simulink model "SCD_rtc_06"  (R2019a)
settings: configuration reference "configurationSettings" (kept in a data dictionary, not in this file)
undefined symbols (not defined in the file or in its folder): algo_demo1_fp, SCDnode06params

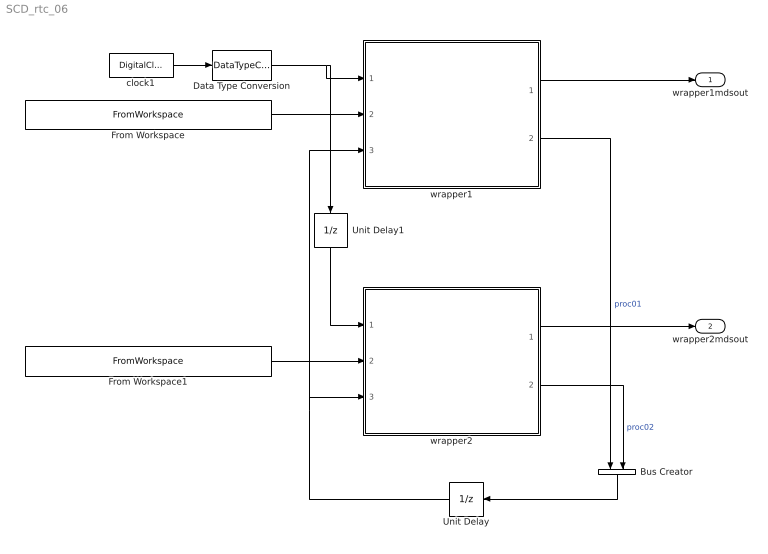
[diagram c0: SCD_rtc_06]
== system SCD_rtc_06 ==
  Bus Creator : BusCreator  Inputs=2
  Data Type Conversion : DataTypeConversion  OutDataTypeStr=single
  From Workspace : FromWorkspace  VariableName=SCDsimdata.SCDnode0601_simdata.wavegen  OutDataTypeStr=Bus: WG0601bus  SampleTime=SCDnode06params.timing.dt  Interpolate=off  OutputAfterFinalValue=Holding final value
  From Workspace1 : FromWorkspace  VariableName=SCDsimdata.SCDnode0602_simdata.wavegen  OutDataTypeStr=Bus: WG0602bus  SampleTime=SCDnode06params.timing.dt  Interpolate=off  OutputAfterFinalValue=Holding final value
  Unit Delay : UnitDelay  SampleTime=-1  HasFrameUpgradeWarning=on
  Unit Delay1 : UnitDelay  SampleTime=-1  HasFrameUpgradeWarning=on
  clock1 : DigitalClock  SampleTime=algo_demo1_fp.timing.dt
  wrapper1 : ModelReference  ModelNameDialog=SCDwrap_demo1.slx  SimulationMode=Normal  ModelReferenceVersion=1.24
  wrapper2 : ModelReference  ModelNameDialog=SCDwrap_demo2.slx  SimulationMode=Normal  ModelReferenceVersion=1.14
  wrapper1mdsout : Outport  OutDataTypeStr=Bus: mdsout01
  wrapper2mdsout : Outport  Port=2  OutDataTypeStr=Bus: mdsout02
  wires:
  wrapper1/1 -> wrapper1mdsout/1
  wrapper2/1 -> wrapper2mdsout/1
  wrapper1/2 -> Bus Creator/1  "proc01"
  wrapper2/2 -> Bus Creator/2  "proc02"
  Bus Creator/1 -> Unit Delay/1
  Unit Delay/1 -> wrapper2/3, wrapper1/3
  From Workspace/1 -> wrapper1/2
  clock1/1 -> Data Type Conversion/1
  Data Type Conversion/1 -> wrapper1/1, Unit Delay1/1
  From Workspace1/1 -> wrapper2/2
  Unit Delay1/1 -> wrapper2/1
